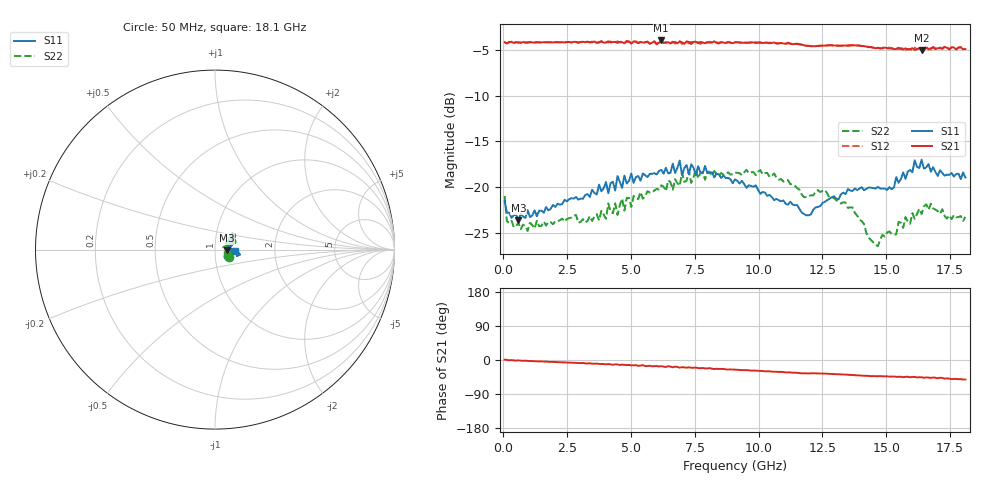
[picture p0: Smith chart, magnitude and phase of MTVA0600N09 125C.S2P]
! Network Analyzer HP8720D.06.14 Serial No. US36140669
!  7 Jul 2005  06:55:32
! Frequency  S11  S21  S12  S22
# HZ  S  DB R 50
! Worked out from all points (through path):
!   201 points, 50 MHz to 18.1 GHz, reference 50 ohm
!   highest |S21| = -3.90 dB at 6.187 GHz (marker M1); lowest = -4.9 dB at 16.39 GHz (marker M2)
!   group delay of S21, straight-line fit = 8.03 ps
!   lowest |S11| = -23.7 dB at 591.5 MHz (marker M3), VSWR 1.14, Z = 57 - j0.344 ohm
!   |S11| at or under -10 dB: start of sweep to end of sweep
!   |S22| runs from -26.5 to -18.0 dB; largest |S21 - S12| = 0.023
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5e7  -21.54 -26.3  -4.10 1.0  -4.10 1.0  -20.99 -27.2
1.4025e8  -22.82 -15.0  -4.23 0.1  -4.21 -0.0  -23.75 -14.8
5.915e8  -23.65 -2.6  -4.09 -0.9  -4.17 -1.2  -23.93 0.6
3.1185e9  -21.29 13.6  -4.04 -7.8  -4.09 -8.1  -23.53 18.8
4.47225e9  -18.80 20.4  -4.18 -11.8  -3.99 -12.0  -23.07 31.2
6.09675e9  -18.25 32.4  -4.16 -17.0  -4.05 -17.1  -20.26 32.8
6.187e9  -18.11 36.1  -3.90 -16.4  -4.00 -16.4  -19.81 31.7
6.7285e9  -18.46 38.9  -4.06 -17.4  -4.25 -17.5  -19.14 29.9
6.909e9  -17.09 38.1  -4.01 -20.2  -3.99 -19.0  -19.87 30.8
6.99925e9  -18.70 37.6  -4.10 -19.0  -4.29 -19.9  -18.41 32.9
7.36025e9  -17.49 34.5  -4.29 -20.4  -4.05 -20.5  -19.54 36.3
7.54075e9  -18.70 35.9  -4.04 -19.8  -4.06 -22.0  -18.04 35.4
7.90175e9  -17.69 40.0  -4.21 -22.3  -4.06 -21.5  -19.20 30.7
9.075e9  -19.16 38.4  -4.11 -25.6  -4.09 -25.8  -18.44 24.7
1.060925e10  -21.44 27.6  -4.12 -31.0  -4.20 -31.3  -18.51 19.5
1.21435e10  -22.47 13.5  -4.54 -35.0  -4.49 -35.3  -20.91 31.3
1.367775e10  -20.45 -8.8  -4.42 -39.5  -4.42 -39.7  -22.25 20.1
1.46705e10  -19.98 -15.7  -4.71 -42.9  -4.70 -42.8  -26.50 15.5
1.512175e10  -20.01 -12.6  -4.80 -43.8  -4.68 -43.9  -24.88 9.7
1.638525e10  -16.99 -12.3  -4.95 -45.5  -4.71 -45.7  -22.96 1.8
1.674625e10  -18.31 -13.4  -4.76 -47.4  -4.91 -47.4  -21.83 -7.6
1.81e10  -18.96 -3.4  -4.85 -51.4  -4.88 -51.7  -23.28 -19.7
